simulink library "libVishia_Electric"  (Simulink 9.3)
settings: Solver=ode45  StartTime=0.0  StopTime=10.0  RelTol=1e-3  EnableMultiTasking=on
undefined symbols (not defined in the file or in its folder): C, Cp, Cs, ctRange, enable_Diode, fnom, gstart, Inom, Lline, n0, n2, nDamping, nHDamping, nIH, nIq, nLs, nPdamping, nRs, pWCstart, Rline, Rps, Rs, RsC, Tmech, Ts, TstepHw, Unom, xh
libraries: powerlib x111, libVishia_Conv x15, libVishia_Ctrl x6, $bdroot x2, lib_T1Blocks_FB x2, Lib_EnvA x1, lib_AngleBlocks x1
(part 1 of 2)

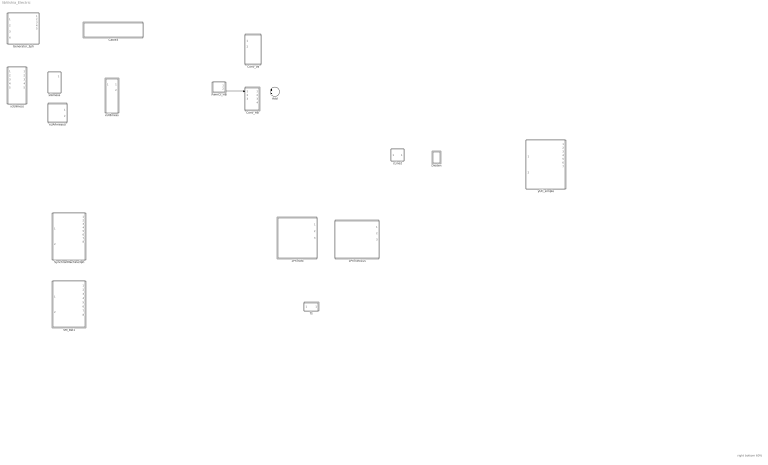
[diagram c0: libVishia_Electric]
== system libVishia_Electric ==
  note: right bottom 60%
  1PhTrafo : Subsystem
  1PhTrafo1us : Subsystem
  Add : Sum
  Cable3 : Subsystem
  Conv_HB : Subsystem
  Conv_Va : Subsystem
  Dioden : Subsystem
  Generator_3ph : Subsystem
  PwmCt_HB : Subsystem
  SM_Bel1 : Subsystem
  SynchronMachine3ph : Subsystem
  Ts : Subsystem
  cLine2 : Subsystem
  x3UImess : Subsystem
  xIAmess : Subsystem
  xUAFmeasU : Subsystem
  xUI3mess : Subsystem
  yUC_simple : Subsystem
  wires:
  PwmCt_HB/2(Out3) -> Conv_HB/1(In2)

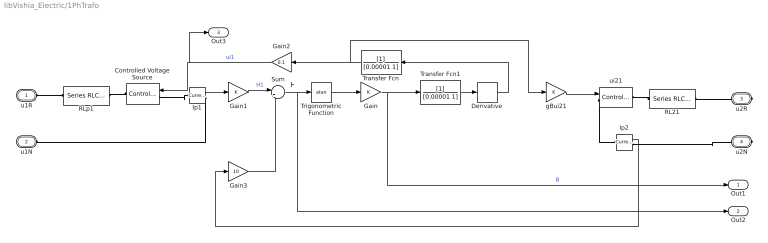
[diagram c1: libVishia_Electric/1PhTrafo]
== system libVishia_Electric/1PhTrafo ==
  note: H
  Controlled Voltage Source : powerlib/Electrical Sources/Controlled Voltage Source  Initialize=on  Source_Type=AC  Amplitude=0  Phase=0  Frequency=0  Measurements=None
  Derivative : Derivative
  Gain : Gain
  Gain1 : Gain
  Gain2 : Gain  Gain=0.1
  Gain3 : Gain  Gain=10
  Ip1 : powerlib/Measurements/Current Measurement  PhasorSimulation=off  OutputType=Complex  PSBequivalent=0
  Ip2 : powerlib/Measurements/Current Measurement  PhasorSimulation=off  OutputType=Complex  PSBequivalent=0
  RL21 : powerlib/Elements/Series RLC Branch  LConnTagsString=__new0  RConnTagsString=__new0  BranchType=RL  Resistance=1  Inductance=1e-3  SetiL0=off  InitialCurrent=0  Capacitance=1e-6  Setx0=off  InitialVoltage=0  Measurements=None
  RLp1 : powerlib/Elements/Series RLC Branch  LConnTagsString=__new0  RConnTagsString=__new0  BranchType=RL  Resistance=0.1  Inductance=0.0001  SetiL0=off  InitialCurrent=0  Capacitance=1e-6  Setx0=off  InitialVoltage=0  Measurements=None
  Sum : Sum  Inputs=|++
  Transfer Fcn : TransferFcn  Denominator=[0.00001 1]
  Transfer Fcn1 : TransferFcn  Denominator=[0.00001 1]
  Trigonometric Function : Trigonometry  Operator=atan
  gBui21 : Gain
  ui21 : powerlib/Electrical Sources/Controlled Voltage Source  Initialize=on  Source_Type=AC  Amplitude=0  Phase=0  Frequency=0  Measurements=None
  u1R : PMIOPort  Tag=PMCPort  Side=Left
  u1N : PMIOPort  Tag=PMCPort  Port=2  Side=Left
  u2R : PMIOPort  Tag=PMCPort  Port=3  Side=Right
  u2N : PMIOPort  Tag=PMCPort  Port=4  Side=Right
  Out1 : Outport
  Out2 : Outport  Port=2
  Out3 : Outport  Port=3
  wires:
  Trigonometric Function/1 -> Gain/1
  Gain/1 -> Transfer Fcn1/1, Out1/1  "B"
  gBui21/1 -> ui21/1
  Gain2/1 -> Out3/1, Controlled Voltage Source/1  "ui1"
  Derivative/1 -> Transfer Fcn/1
  Ip1/1 -> Gain1/1
  Transfer Fcn/1 -> gBui21/1, Gain2/1
  Gain1/1 -> Sum/1  "H1"
  Sum/1 -> Out2/1, Trigonometric Function/1
  Gain3/1 -> Sum/2
  Ip2/1 -> Gain3/1
  Transfer Fcn1/1 -> Derivative/1
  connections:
  u2R/RConn1 -- RL21/RConn1
  RLp1/RConn1 -- Controlled Voltage Source/RConn1
  Ip1/LConn1 -- Controlled Voltage Source/LConn1
  RLp1/LConn1 -- u1R/RConn1
  RL21/LConn1 -- ui21/RConn1
  Ip1/RConn1 -- u1N/RConn1
  ui21/LConn1 -- Ip2/LConn1
  u2N/RConn1 -- Ip2/RConn1

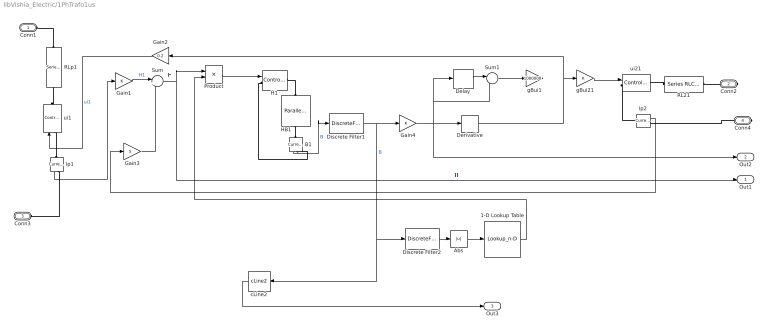
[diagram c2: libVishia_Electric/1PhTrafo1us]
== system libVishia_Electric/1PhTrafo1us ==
  note: H
  1-D Lookup Table : Lookup_n-D  NumberOfTableDimensions=1  BreakpointsForDimension1=[0 1 2 3 4 5]  Table="[1.0 0.9 0.7 0.3 0.15 0.05  ]"  InternalRulePriority=Speed  RndMeth=Simplest
  Abs : Abs
  B1 : powerlib/Measurements/Current Measurement  PhasorSimulation=off  OutputType=Complex  PSBequivalent=0
  Delay : Delay  DelayLength=1
  Derivative : Derivative
  Discrete Filter1 : DiscreteFilter  Denominator=[1 0.00001]
  Discrete Filter2 : DiscreteFilter  Denominator=[1 0.0001]
  Gain1 : Gain
  Gain2 : Gain  Gain=0.2
  Gain3 : Gain  Gain=5
  Gain4 : Gain
  H1 : powerlib/Electrical Sources/Controlled Voltage Source  Initialize=on  Source_Type=AC  Amplitude=0  Phase=0  Frequency=0  Measurements=None
  HB1 : powerlib/Elements/Parallel RLC Branch  LConnTagsString=a  RConnTagsString=__new0  BranchType=R  Resistance=1  Inductance=1e-3  SetiL0=off  InitialCurrent=0  Capacitance=1e-6  Setx0=off  InitialVoltage=0  Measurements=None
  Ip1 : powerlib/Measurements/Current Measurement  PhasorSimulation=off  OutputType=Complex  PSBequivalent=0
  Ip2 : powerlib/Measurements/Current Measurement  PhasorSimulation=off  OutputType=Complex  PSBequivalent=0
  Product : Product
  RL21 : powerlib/Elements/Series RLC Branch  LConnTagsString=__new0  RConnTagsString=__new0  BranchType=RL  Resistance=1  Inductance=1e-3  SetiL0=off  InitialCurrent=0  Capacitance=1e-6  Setx0=off  InitialVoltage=0  Measurements=None
  RLp1 : powerlib/Elements/Series RLC Branch  LConnTagsString=__new0  RConnTagsString=__new0  BranchType=RL  Resistance=0.1  Inductance=0.0001  SetiL0=off  InitialCurrent=0  Capacitance=1e-6  Setx0=off  InitialVoltage=0  Measurements=None
  Sum : Sum  Inputs=|++
  Sum1 : Sum  Inputs=|-+
  cLine2 : Lib_EnvA/cLine2  n0=1  xh=5  n2=0.05
  gBui1 : Gain  Gain=1000000
  gBui21 : Gain
  ui1 : powerlib/Electrical Sources/Controlled Voltage Source  Initialize=on  Source_Type=AC  Amplitude=0  Phase=0  Frequency=0  Measurements=None
  ui21 : powerlib/Electrical Sources/Controlled Voltage Source  Initialize=on  Source_Type=AC  Amplitude=0  Phase=0  Frequency=0  Measurements=None
  Conn1 : PMIOPort  Side=Left
  Conn2 : PMIOPort  Port=2  Side=Right
  Conn3 : PMIOPort  Port=3  Side=Left
  Conn4 : PMIOPort  Port=4  Side=Right
  Out1 : Outport
  Out2 : Outport  Port=2
  Out3 : Outport  Port=3
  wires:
  Abs/1 -> 1-D Lookup Table/1
  Discrete Filter2/1 -> Abs/1
  cLine2/1 -> Out3/1
  1-D Lookup Table/1 -> Product/2
  Gain4/1 -> Derivative/1, Out2/1, Sum1/2, Delay/1
  Gain2/1 -> ui1/1  "ui1"
  Ip2/1 -> Gain3/1
  Gain3/1 -> Sum/2
  Ip1/1 -> Gain1/1
  B1/1 -> Discrete Filter1/1  "B"
  gBui21/1 -> ui21/1
  Sum/1 -> Product/1, Out1/1  "H"
  Gain1/1 -> Sum/1  "H1"
  Sum1/1 -> gBui1/1
  Delay/1 -> Sum1/1
  Discrete Filter1/1 -> Gain4/1, cLine2/1, Discrete Filter2/1  "B"
  Derivative/1 -> Gain2/1, gBui21/1
  Product/1 -> H1/1
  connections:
  ui21/LConn1 -- Ip2/LConn1
  RLp1/RConn1 -- ui1/RConn1
  RLp1/LConn1 -- Conn1/RConn1
  Conn4/RConn1 -- Ip2/RConn1
  Ip1/RConn1 -- Conn3/RConn1
  RL21/RConn1 -- Conn2/RConn1
  RL21/LConn1 -- ui21/RConn1
  Ip1/LConn1 -- ui1/LConn1
  HB1/LConn1 -- H1/RConn1
  HB1/RConn1 -- B1/LConn1
  H1/LConn1 -- B1/RConn1

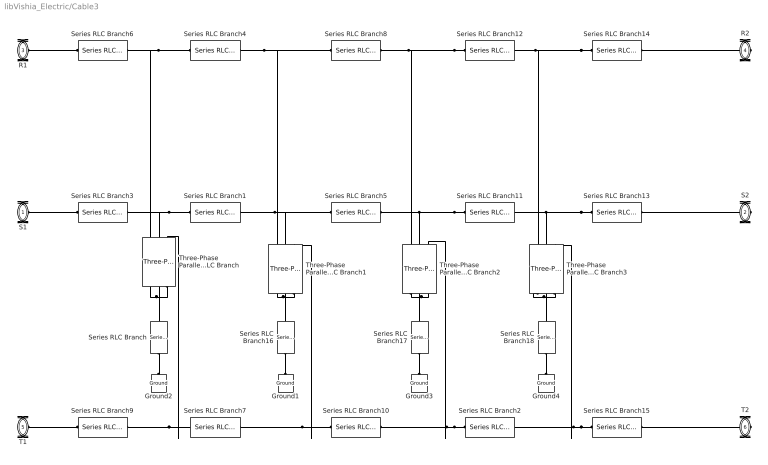
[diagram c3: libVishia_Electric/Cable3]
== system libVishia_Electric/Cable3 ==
  Ground{1..4} (4 alike) : powerlib/Elements/Ground  LConnTagsString=a
  Series RLC Branch{,16..18} (4 alike) : powerlib/Elements/Series RLC Branch  LConnTagsString=__new0  RConnTagsString=__new0  BranchType=R  Resistance=RsC  Inductance=1e-3  SetiL0=off  InitialCurrent=0  Capacitance=1e-6  Setx0=off  InitialVoltage=0  Measurements=None
  Series RLC Branch{1..2,4..5,7..8,10..12} (9 alike) : powerlib/Elements/Series RLC Branch  LConnTagsString=__new0  RConnTagsString=__new0  BranchType=RL  Resistance=Rline/4  Inductance=Lline/4  SetiL0=off  InitialCurrent=0  Capacitance=C  Setx0=off  InitialVoltage=0  Measurements=None
  Series RLC Branch{3,6,9,13..15} (6 alike) : powerlib/Elements/Series RLC Branch  LConnTagsString=__new0  RConnTagsString=__new0  BranchType=RL  Resistance=Rline/8  Inductance=Lline/8  SetiL0=off  InitialCurrent=0  Capacitance=C  Setx0=off  InitialVoltage=0  Measurements=None
  Three-Phase Parallel RLC Branch{,1..3} (4 alike) : powerlib/Elements/Three-Phase Parallel RLC Branch  LConnTagsString=A|B|C  RConnTagsString=A|B|C  BranchType=RC  Resistance=Rs/4  Inductance=1e-3  Capacitance=Cs/4  Measurements=None
  S1 : PMIOPort  Side=Left
  S2 : PMIOPort  Port=2  Side=Right
  R1 : PMIOPort  Port=3  Side=Left
  R2 : PMIOPort  Port=4  Side=Right
  T1 : PMIOPort  Port=5  Side=Left
  T2 : PMIOPort  Port=6  Side=Right
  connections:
  Three-Phase Parallel RLC Branch2/RConn1 -- Three-Phase Parallel RLC Branch2/RConn2 -- Series RLC Branch17/LConn1 -- Three-Phase Parallel RLC Branch2/RConn3
  S1/RConn1 -- Series RLC Branch3/RConn1
  Series RLC Branch1/RConn1 -- Three-Phase Parallel RLC Branch/LConn2 -- Series RLC Branch3/LConn1
  Series RLC Branch4/RConn1 -- Three-Phase Parallel RLC Branch/LConn1 -- Series RLC Branch6/LConn1
  R1/RConn1 -- Series RLC Branch6/RConn1
  Series RLC Branch9/LConn1 -- Three-Phase Parallel RLC Branch/LConn3 -- Series RLC Branch7/RConn1
  T1/RConn1 -- Series RLC Branch9/RConn1
  Series RLC Branch4/LConn1 -- Three-Phase Parallel RLC Branch1/LConn1 -- Series RLC Branch8/RConn1
  Series RLC Branch1/LConn1 -- Three-Phase Parallel RLC Branch1/LConn2 -- Series RLC Branch5/RConn1
  Series RLC Branch7/LConn1 -- Three-Phase Parallel RLC Branch1/LConn3 -- Series RLC Branch10/RConn1
  Series RLC Branch12/RConn1 -- Series RLC Branch8/LConn1 -- Three-Phase Parallel RLC Branch2/LConn1
  Series RLC Branch11/RConn1 -- Series RLC Branch5/LConn1 -- Three-Phase Parallel RLC Branch2/LConn2
  Series RLC Branch2/RConn1 -- Series RLC Branch10/LConn1 -- Three-Phase Parallel RLC Branch2/LConn3
  Series RLC Branch14/RConn1 -- Series RLC Branch12/LConn1 -- Three-Phase Parallel RLC Branch3/LConn1
  Series RLC Branch13/RConn1 -- Series RLC Branch11/LConn1 -- Three-Phase Parallel RLC Branch3/LConn2
  Series RLC Branch15/RConn1 -- Series RLC Branch2/LConn1 -- Three-Phase Parallel RLC Branch3/LConn3
  R2/RConn1 -- Series RLC Branch14/LConn1
  S2/RConn1 -- Series RLC Branch13/LConn1
  T2/RConn1 -- Series RLC Branch15/LConn1
  Three-Phase Parallel RLC Branch/RConn3 -- Series RLC Branch/LConn1 -- Three-Phase Parallel RLC Branch/RConn1 -- Three-Phase Parallel RLC Branch/RConn2
  Three-Phase Parallel RLC Branch1/RConn3 -- Series RLC Branch16/LConn1 -- Three-Phase Parallel RLC Branch1/RConn1 -- Three-Phase Parallel RLC Branch1/RConn2
  Three-Phase Parallel RLC Branch3/RConn3 -- Three-Phase Parallel RLC Branch3/RConn2 -- Series RLC Branch18/LConn1 -- Three-Phase Parallel RLC Branch3/RConn1
  Series RLC Branch/RConn1 -- Ground2/LConn1
  Series RLC Branch16/RConn1 -- Ground1/LConn1
  Series RLC Branch17/RConn1 -- Ground3/LConn1
  Series RLC Branch18/RConn1 -- Ground4/LConn1

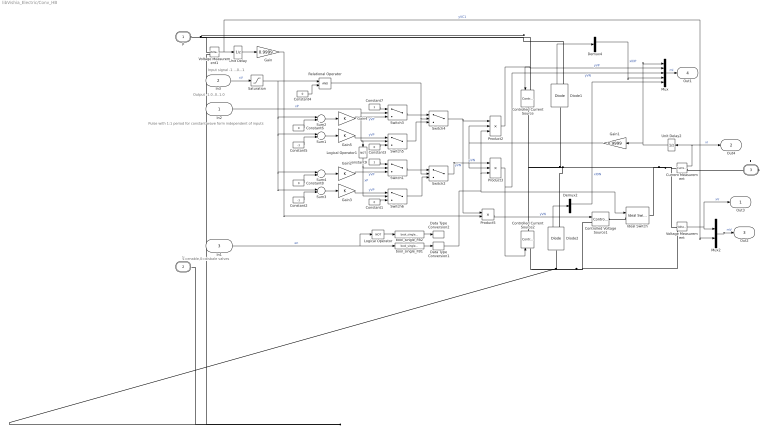
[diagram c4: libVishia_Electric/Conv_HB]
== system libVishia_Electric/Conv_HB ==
  note: Pulse with 1:1 period for constant wave form independent of inputs
  note: Input signal -1 ...0...1
  note: 1=enable,0=disbale valves
  note: Output -1.0..0..1.0
  In2 : Inport
  In3 : Inport  Port=2  OutDataTypeStr=single
  In1 : Inport  Port=3
  Constant{1,3..4,6,8} (5 alike) : Constant  Value=0
  Constant2 : Constant  Value=-1
  Constant5 : Constant  Value=-1
  Constant7 : Constant
  Constant9 : Constant
  Controlled Current Source : powerlib/Electrical Sources/Controlled Current Source  Initialize=on  Source_Type=AC  Amplitude=0  Phase=0  Frequency=0  Measurements=None
  Controlled Current Source2 : powerlib/Electrical Sources/Controlled Current Source  Initialize=on  Source_Type=AC  Amplitude=0  Phase=0  Frequency=0  Measurements=None
  Controlled Voltage Source1 : powerlib/Electrical Sources/Controlled Voltage Source  Initialize=on  Source_Type=AC  Amplitude=0  Phase=0  Frequency=0  Measurements=None
  Current Measurement : powerlib/Measurements/Current Measurement  PhasorSimulation=off  OutputType=Complex  PSBequivalent=0
  Data Type Conversion1 : DataTypeConversion  OutDataTypeStr=double
  Data Type Conversion2 : DataTypeConversion  OutDataTypeStr=double
  Demux2 : Demux  Outputs=2
  Demux4 : Demux  Outputs=2
  Diode1 : powerlib/Power Electronics/Diode  Ron=0.001  Lon=0  Vf=0.8  IC=0  UseSnubber=0  Rs=500  Cs=250e-9  Measurements=on
  Diode2 : powerlib/Power Electronics/Diode  Ron=0.001  Lon=0  Vf=0.8  IC=0  UseSnubber=0  Rs=500  Cs=250e-9  Measurements=on
  Gain : Gain  Gain=0.9999
  Gain1 : Gain  Gain=0.9999
  Gain{2..5} (4 alike) : Gain
  Ideal Switch : powerlib/Power Electronics/Ideal Switch  Ron=0.001  Lon=0  IC=0  Rs=1e5  Cs=inf  Measurements=off
  Logical Operator : Logic  Operator=NOT  IconShape=distinctive  AllPortsSameDT=off  OutDataTypeStr=boolean
  Logical Operator1 : Logic  Operator=NOT  IconShape=distinctive  AllPortsSameDT=off  OutDataTypeStr=boolean
  Mux : Mux  Inputs=5
  Mux2 : Mux  Inputs=2
  Product2 : Product  Inputs=3
  Product3 : Product  Inputs=3
  Product5 : Product
  Relational Operator : RelationalOperator  OutDataTypeStr=boolean  RndMeth=Simplest
  Saturation : Saturate  UpperLimit=1.0  LowerLimit=-1.0
  Sum{1..4} (4 alike) : Sum  Inputs=|+-
  Switch{1..6} (6 alike) : Switch  Criteria=u2 ~= 0
  Unit Delay : UnitDelay  SampleTime=-1  HasFrameUpgradeWarning=on
  Unit Delay2 : UnitDelay  SampleTime=-1  HasFrameUpgradeWarning=on
  Voltage Measurement : powerlib/Measurements/Voltage Measurement  PhasorSimulation=off  OutputType=Complex  PSBequivalent=0
  Voltage Measurement1 : powerlib/Measurements/Voltage Measurement  PhasorSimulation=off  OutputType=Complex  PSBequivalent=0
  bool_single_FB1 : libVishia_Conv/bool_single_FB  hi=1  lo=0
  bool_single_FB2 : libVishia_Conv/bool_single_FB  hi=1  lo=0
  P : PMIOPort  Tag=PMCPort  Side=Left
  N : PMIOPort  Tag=PMCPort  Port=2  Side=Left
  L : PMIOPort  Tag=PMCPort  Port=3  Side=Right
  Out3 : Outport  OutDataTypeStr=double
  Out4 : Outport  Port=2  OutDataTypeStr=double
  Out2 : Outport  Port=3  OutDataTypeStr=double
  Out1 : Outport  Port=4  OutDataTypeStr=double
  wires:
  Diode2/1 -> Demux2/1
  Diode1/1 -> Demux4/1
  Data Type Conversion1/1 -> Product2/3, Product3/3, Ideal Switch/1
  bool_single_FB1/1 -> Data Type Conversion1/1
  In1/1 -> Logical Operator/1, bool_single_FB1/1  "en"
  Switch3/1 -> Switch4/1
  Constant7/1 -> Switch3/1
  Switch4/1 -> Product5/1, Product2/1  "yVN"
  Sum2/1 -> Gain4/1
  Constant6/1 -> Sum2/2
  Constant5/1 -> Sum1/2
  Sum1/1 -> Gain5/1
  Constant4/1 -> Relational Operator/2
  Relational Operator/1 -> Switch2/2, Switch4/2
  Switch5/1 -> Switch4/3
  Constant3/1 -> Switch5/3
  Gain5/1 -> Switch5/1  "yVP"
  Gain4/1 -> Switch3/3  "yVP"
  Product3/1 -> Controlled Current Source2/1, Mux/3  "yVN"
  Product2/1 -> Controlled Current Source/1, Mux/2  "yVP"
  Product5/1 -> Controlled Voltage Source1/1  "yVN"
  Voltage Measurement1/1 -> Unit Delay/1, Mux2/2  "yVC1"
  In2/1 -> Logical Operator1/1, Switch5/2, Switch3/2  "xP"
  Gain/1 -> Product5/2
  Demux4/1 -> Mux/4  "xIDP"
  Demux2/1 -> Mux/5  "xIDN"
  Mux/1 -> Out1/1  "mI"
  Mux2/1 -> Out2/1  "mV"
  Current Measurement/1 -> Out4/1, Unit Delay2/1  "xI"
  Voltage Measurement/1 -> Out3/1, Mux2/1  "xV"
  Gain1/1 -> Product2/2, Product3/2
  Unit Delay2/1 -> Mux/1, Gain1/1
  Unit Delay/1 -> Gain/1
  bool_single_FB2/1 -> Data Type Conversion2/1
  Logical Operator/1 -> bool_single_FB2/1
  In3/1 -> Saturation/1  "xV"
  Constant2/1 -> Sum3/2
  Constant1/1 -> Switch6/3
  Logical Operator1/1 -> Switch1/2, Switch6/2  "xP"
  Gain2/1 -> Switch1/3  "yVP"
  Sum3/1 -> Gain3/1
  Constant8/1 -> Sum4/2
  Switch1/1 -> Switch2/1
  Sum4/1 -> Gain2/1
  Constant9/1 -> Switch1/1
  Switch6/1 -> Switch2/3
  Gain3/1 -> Switch6/1  "yVP"
  Switch2/1 -> Product3/1  "yVN"
  Saturation/1 -> Sum3/1, Sum4/1, Sum1/1, Sum2/1, Relational Operator/1
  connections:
  Ideal Switch/LConn1 -- Controlled Voltage Source1/RConn1
  Controlled Current Source/LConn1 -- Diode1/RConn1 -- P/RConn1 -- Voltage Measurement1/LConn1
  Controlled Current Source2/LConn1 -- N/RConn1 -- Voltage Measurement1/LConn2 -- Diode2/LConn1 -- Controlled Voltage Source1/LConn1 -- Voltage Measurement/LConn2
  Voltage Measurement/LConn1 -- Current Measurement/LConn1 -- Ideal Switch/RConn1 -- Diode1/LConn1 -- Controlled Current Source/RConn1 -- Controlled Current Source2/RConn1 -- Diode2/RConn1
  Current Measurement/RConn1 -- L/RConn1

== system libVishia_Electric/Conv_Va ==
  In1 : Inport
  In2 : Inport  Port=2
  Diode2 : powerlib/Power Electronics/Diode  Ron=0.001  Lon=0  Vf=0.8  IC=0  UseSnubber=0  Rs=500  Cs=250e-9  Measurements=on
  Diode3 : powerlib/Power Electronics/Diode  Ron=0.001  Lon=0  Vf=0.8  IC=0  UseSnubber=0  Rs=500  Cs=250e-9  Measurements=on
  Ideal Switch : powerlib/Power Electronics/Ideal Switch  Ron=0.001  Lon=0  IC=0  Rs=1e5  Cs=inf  Measurements=on
  Ideal Switch1 : powerlib/Power Electronics/Ideal Switch  Ron=0.001  Lon=0  IC=0  Rs=1e5  Cs=inf  Measurements=on
  Series RLC Branch : powerlib/Elements/Series RLC Branch  LConnTagsString=__new0  RConnTagsString=__new0  BranchType=RC  Resistance=Rps  Inductance=1e-3  SetiL0=off  InitialCurrent=0  Capacitance=Cp  Setx0=off  InitialVoltage=0  Measurements=None
  Series RLC Branch1 : powerlib/Elements/Series RLC Branch  LConnTagsString=__new0  RConnTagsString=__new0  BranchType=RC  Resistance=Rps  Inductance=1e-3  SetiL0=off  InitialCurrent=0  Capacitance=Cp  Setx0=off  InitialVoltage=0  Measurements=None
  bool2single1 : libVishia_Conv/bool_single_FB  hi=1.0  lo=0
  bool2single3 : libVishia_Conv/bool_single_FB  hi=1.0  lo=0
  P : PMIOPort  Tag=PMCPort  Side=Left
  N : PMIOPort  Tag=PMCPort  Port=2  Side=Left
  L : PMIOPort  Tag=PMCPort  Port=3  Side=Right
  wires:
  In1/1 -> bool2single3/1  "H"
  In2/1 -> bool2single1/1  "L"
  bool2single3/1 -> Ideal Switch/1
  bool2single1/1 -> Ideal Switch1/1
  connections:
  Ideal Switch/RConn1 -- Series RLC Branch1/LConn1 -- L/RConn1 -- Series RLC Branch/RConn1 -- Diode3/RConn1 -- Diode2/LConn1 -- Ideal Switch1/LConn1
  N/RConn1 -- Series RLC Branch1/RConn1 -- Diode3/LConn1 -- Ideal Switch1/RConn1
  P/RConn1 -- Series RLC Branch/LConn1 -- Diode2/RConn1 -- Ideal Switch/LConn1

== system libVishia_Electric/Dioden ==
  Breaker : powerlib/Elements/Breaker  InitialState=0  SwitchingTimes="[ 1/60  5/60 ]"  External=on  BreakerResistance=0.0000001  SnubberResistance=inf  SnubberCapacitance=1e-6  Measurements=None  MoreParameters=off  NoBreakLoop=off
  Constant : Constant  Value=enable_Diode  OutDataTypeStr=int32
  Diode : powerlib/Power Electronics/Diode  Ron=0.0001  Lon=0  Vf=Vf_Diode  IC=0  UseSnubber=off  Rs=inf  Cs=0  Measurements=off
  Diode3 : powerlib/Power Electronics/Diode  Ron=0.0001  Lon=0  Vf=Vf_Diode  IC=0  UseSnubber=off  Rs=inf  Cs=0  Measurements=off
  Logical Operator : Logic  Operator=NOT  AllPortsSameDT=off  OutDataTypeStr=boolean
  Series RLC Branch : powerlib/Elements/Series RLC Branch  LConnTagsString=__new0  RConnTagsString=__new0  BranchType=R  Resistance=10000  Inductance=1e-3  SetiL0=off  InitialCurrent=0  Capacitance=1e-6  Setx0=off  InitialVoltage=0  Measurements=None
  in : PMIOPort  Tag=PMCPort  Side=Left
  out : PMIOPort  Tag=PMCPort  Port=2  Side=Right
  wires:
  Logical Operator/1 -> Breaker/1
  Constant/1 -> Logical Operator/1
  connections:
  Series RLC Branch/LConn1 -- Diode3/RConn1 -- in/RConn1 -- Breaker/LConn1 -- Diode/LConn1
  Series RLC Branch/RConn1 -- Diode/RConn1 -- out/RConn1 -- Breaker/RConn1 -- Diode3/LConn1

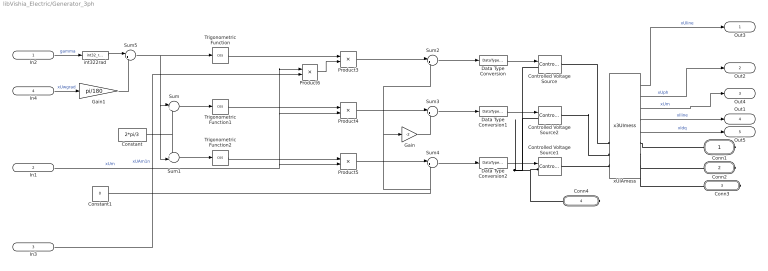
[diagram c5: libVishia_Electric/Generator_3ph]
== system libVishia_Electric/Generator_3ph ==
  In2 : Inport  OutDataTypeStr=int32
  In1 : Inport  Port=2  OutDataTypeStr=single  PortDimensions=1
  In3 : Inport  Port=3  OutDataTypeStr=single  PortDimensions=1
  In4 : Inport  Port=4  OutDataTypeStr=single  PortDimensions=1
  Constant : Constant  Value=2*pi/3  OutDataTypeStr=single
  Constant1 : Constant  Value=0
  Controlled Voltage Source : powerlib/Electrical Sources/Controlled Voltage Source  Initialize=on  Source_Type=AC  Amplitude=0  Phase=0  Frequency=0  Measurements=None
  Controlled Voltage Source1 : powerlib/Electrical Sources/Controlled Voltage Source  Initialize=on  Source_Type=AC  Amplitude=0  Phase=0  Frequency=0  Measurements=None
  Controlled Voltage Source2 : powerlib/Electrical Sources/Controlled Voltage Source  Initialize=on  Source_Type=AC  Amplitude=0  Phase=0  Frequency=0  Measurements=None
  Data Type Conversion : DataTypeConversion
  Data Type Conversion1 : DataTypeConversion
  Data Type Conversion2 : DataTypeConversion
  Gain : Gain  Gain=-2
  Gain1 : Gain  Gain=pi/180
  Product{3..6} (4 alike) : Product
  Sum : Sum  Inputs=|+-
  Sum1 : Sum  Inputs=++|
  Sum{2..5} (4 alike) : Sum  Inputs=|++
  Trigonometric Function : Trigonometry  Operator=cos
  Trigonometric Function1 : Trigonometry  Operator=cos
  Trigonometric Function2 : Trigonometry  Operator=cos
  int322rad : libVishia_Conv/int32_rad_FB  SystemSampleTime=-1
  xUIAmess : $bdroot/x3UImess  SystemSampleTime=-1
  Conn1 : PMIOPort  Side=Right
  Conn2 : PMIOPort  Port=2  Side=Right
  Conn3 : PMIOPort  Port=3  Side=Right
  Conn4 : PMIOPort  Port=4  Side=Right
  Out3 : Outport  OutDataTypeStr=single  PortDimensions=3
  Out2 : Outport  Port=2  OutDataTypeStr=single  PortDimensions=3
  Out4 : Outport  Port=3  OutDataTypeStr=single  PortDimensions=1
  Out1 : Outport  Port=4  OutDataTypeStr=single  PortDimensions=3
  Out5 : Outport  Port=5  OutDataTypeStr=single  PortDimensions=1
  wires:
  Constant/1 -> Sum1/1, Sum/2
  Sum1/1 -> Trigonometric Function2/1
  Sum/1 -> Trigonometric Function1/1
  Sum5/1 -> Sum1/2, Sum/1, Trigonometric Function/1
  In2/1 -> int322rad/1  "gamma"
  Data Type Conversion/1 -> Controlled Voltage Source/1
  Data Type Conversion1/1 -> Controlled Voltage Source2/1
  Data Type Conversion2/1 -> Controlled Voltage Source1/1
  Product4/1 -> Sum3/1
  Product3/1 -> Sum2/1
  In1/1 -> Product6/1, Product4/2, Product5/2  "xUm"
  Product5/1 -> Sum4/1
  Trigonometric Function/1 -> Product3/1
  Trigonometric Function1/1 -> Product4/1
  Trigonometric Function2/1 -> Product5/1
  Sum2/1 -> Data Type Conversion/1
  Sum3/1 -> Data Type Conversion1/1
  Sum4/1 -> Data Type Conversion2/1
  Constant1/1 -> Gain/1, Sum2/2, Sum4/2
  Gain/1 -> Sum3/2
  Product6/1 -> Product3/2
  In3/1 -> Product6/2  "xUAm1n"
  int322rad/1 -> Sum5/1
  In4/1 -> Gain1/1  "xUwgrad"
  Gain1/1 -> Sum5/2
  xUIAmess/2 -> Out2/1  "xUph"
  xUIAmess/1 -> Out3/1  "xUline"
  xUIAmess/4 -> Out1/1  "xIline"
  xUIAmess/3 -> Out4/1  "xUm"
  xUIAmess/5 -> Out5/1  "xIdq"
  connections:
  Controlled Voltage Source1/LConn1 -- Conn4/RConn1 -- Controlled Voltage Source/LConn1 -- Controlled Voltage Source2/LConn1
  xUIAmess/LConn1 -- Controlled Voltage Source/RConn1
  xUIAmess/LConn2 -- Controlled Voltage Source2/RConn1
  xUIAmess/LConn3 -- Controlled Voltage Source1/RConn1
  xUIAmess/RConn3 -- Conn3/RConn1
  xUIAmess/RConn2 -- Conn2/RConn1
  xUIAmess/RConn1 -- Conn1/RConn1

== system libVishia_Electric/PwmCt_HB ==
  note: counts from 0 t0 ctRange-1 ctRange should be even (able to divide by 2)
  Constant3 : Constant  Value=0  OutDataTypeStr=int16
  Constant4 : Constant  Value=ctRange-1  OutDataTypeStr=int16
  Constant5 : Constant  OutDataTypeStr=int16
  Constant6 : Constant  Value=ctRange/2  OutDataTypeStr=int16
  Relational Operator2 : RelationalOperator  OutDataTypeStr=boolean  RndMeth=Simplest
  Relational Operator7 : RelationalOperator  OutDataTypeStr=boolean  RndMeth=Simplest
  addS_OpC : libVishia_Ctrl/addS_OpC  init=0  Tstep=-1
  Out2 : Outport  OutDataTypeStr=int16
  Out3 : Outport  Port=2  OutDataTypeStr=boolean
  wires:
  Relational Operator7/1 -> addS_OpC/3
  addS_OpC/2 -> Relational Operator2/1, Relational Operator7/1, Out2/1  "yCt"
  Constant6/1 -> Relational Operator2/2
  Constant4/1 -> Relational Operator7/2
  Constant3/1 -> addS_OpC/2
  Constant5/1 -> addS_OpC/1
  Relational Operator2/1 -> Out3/1  "yP"

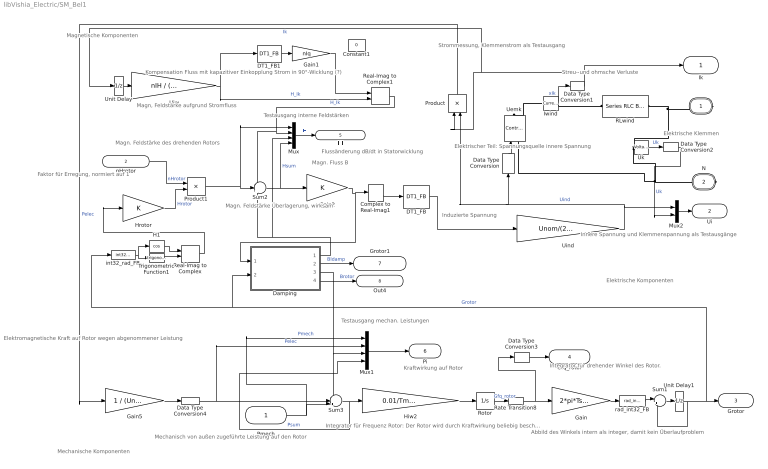
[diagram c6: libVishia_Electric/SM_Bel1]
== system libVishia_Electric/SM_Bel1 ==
  note: Abbild des Winkels intern als integer, damit kein Überlaufproblem
  note: Kompensation Fluss mit kapazitiver Einkopplung Strom in 90°-Wicklung (?)
  note: Testausgang mechan. Leistungen
  note: Mechanische Komponenten
  note: Mechanisch von außen zugeführte Leistung auf den Rotor
  note: Elektromagnetische Kraft auf Rotor wegen abgenommener Leistung
  note: Strommessung, Klemmenstrom als Testausgang
  note: Innere Spannung und Klemmenspannung als Testausgänge
  note: Elektrische Klemmen
  note: Streu- und ohmsche Verluste
  note: Elektrischer Teil: Spannungsquelle innere Spannung
  note: Faktor für Erregung, normiert auf 1
  note: Testausgang interne Feldstärken
  note: Flussänderung dB/dt in Statorwicklung
  note: Magn. Fluss B
  note: Induzierte Spannung
  note: Magn, Feldstärke aufgrund Stromfluss
  note: Magn. Feldstärke Überlagerung, wirksam
  note: Integrator für Frequenz Rotor: Der Rotor wird durch Kraftwirkung beliebig beschleunigt. Reibungsverluste hier unberücksichtigt.
  note: Kraftwirkung auf Rotor
  note: Integrator für drehender Winkel des Rotor.
  note: Magn. Feldstärke des drehenden Rotors
  note: Magnetische Komponenten
  note: Elektrische Komponenten
  Pmech : Inport  OutDataTypeStr=double  PortDimensions=1
  nHrotor : Inport  Port=2  OutDataTypeStr=single  PortDimensions=1
  Complex to Real-Imag1 : ComplexToRealImag
  Constant1 : Constant  Value=0  OutDataTypeStr=single
  DT1_FB : libVishia_Ctrl/DT1_FB  T1=0.0004  Td=1  Tstep=TstepHw
  DT1_FB1 : libVishia_Ctrl/DT1_FB  T1=0.001  Td=0.060/2/pi  Tstep=TstepHw
  Damping : Subsystem
  Data Type Conversion : DataTypeConversion  OutDataTypeStr=double
  Data Type Conversion1 : DataTypeConversion  OutDataTypeStr=single
  Data Type Conversion2 : DataTypeConversion  OutDataTypeStr=single
  Data Type Conversion3 : DataTypeConversion  OutDataTypeStr=single
  Data Type Conversion4 : DataTypeConversion  OutDataTypeStr=double
  Gain : Gain  Gain=2*pi*TstepHw
  Gain1 : Gain  Gain=nIq
  Gain2 : Gain
  Gain5 : Gain  Gain=1 / (Unom*Inom)
  H1 : Trigonometry  Operator=cos
  Hiw : Gain  Gain=nIH / (Inom*sqrt(2))
  Hiw2 : Gain  Gain=0.01/Tmech
  Hrotor : Gain
  Iwind : powerlib/Measurements/Current Measurement  PhasorSimulation=off  OutputType=Complex  PSBequivalent=0
  Mux : Mux
  Mux1 : Mux
  Mux2 : Mux  Inputs=2
  Product : Product
  Product1 : Product
  RLwind : powerlib/Elements/Series RLC Branch  LConnTagsString=__new0  RConnTagsString=__new0  BranchType=RL  Resistance=nRs*Unom/Inom  Inductance=nLs * Unom/Inom / (2*pi*fnom)  SetiL0=off  InitialCurrent=0  Capacitance=1e-6  Setx0=off  InitialVoltage=0  Measurements=None
  Rate Transition8 : RateTransition  Integrity=off  Deterministic=off  OutPortSampleTimeMultiple=16  OutPortSampleTime=TstepHw
  Real-Imag to Complex : RealImagToComplex
  Real-Imag to Complex1 : RealImagToComplex
  Rotor : Integrator  InitialCondition=fnom
  Sum1 : Sum  Inputs=|++
  Sum2 : Sum  Inputs=-++
  Sum3 : Sum  Inputs=--+
  Trigonometric Function1 : Trigonometry
  Uemk : powerlib/Electrical Sources/Controlled Voltage Source  Initialize=on  Source_Type=AC  Amplitude=0  Phase=0  Frequency=0  Measurements=None
  Uind : Gain  Gain=Unom/(2*pi*fnom)*sqrt(2)
  Uk : powerlib/Measurements/Voltage Measurement  PhasorSimulation=off  OutputType=Complex  PSBequivalent=0
  Unit Delay : UnitDelay  SampleTime=-1  HasFrameUpgradeWarning=on
  Unit Delay1 : UnitDelay  InitialCondition=gstart*65536*32768/180  SampleTime=TstepHw  HasFrameUpgradeWarning=on
  int32_rad_FB : libVishia_Conv/int32_rad_FB  SystemSampleTime=-1
  rad_int32_FB : libVishia_Conv/rad_int32_FB  SystemSampleTime=-1
  L : PMIOPort  Tag=PMCPort  Side=Right
  N : PMIOPort  Tag=PMCPort  Port=2  Side=Right
  Ik : Outport  OutDataTypeStr=single  PortDimensions=1
  Ui : Outport  Port=2  PortDimensions=2
  Grotor : Outport  Port=3  OutDataTypeStr=int32  PortDimensions=1
  Gfq_rotor : Outport  Port=4  PortDimensions=1
  Hi : Outport  Port=5  PortDimensions=4
  Pi : Outport  Port=6  OutDataTypeStr=double  PortDimensions=4
  Grotor1 : Outport  Port=7  OutDataTypeStr=single  PortDimensions=3
  Out4 : Outport  Port=8  OutDataTypeStr=single  PortDimensions=1
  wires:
  Damping/2(Out2) -> Grotor1/1  "BIdamp"
  Damping/1(Out1) -> Sum2/3, Mux/3
  Hrotor/1 -> Product1/2  "Hrotor"
  nHrotor/1 -> Product1/1  "nHrotor"
  DT1_FB/2 -> Uind/1
  Hiw2/1 -> Rotor/1
  Data Type Conversion3/1 -> Gfq_rotor/1
  Rate Transition8/1 -> Gain/1, Data Type Conversion3/1
  Mux1/1 -> Pi/1
  Real-Imag to Complex/1 -> Hrotor/1
  Mux2/1 -> Ui/1
  Product/1 -> Gain5/1  "Pelec"
  Data Type Conversion4/1 -> Mux1/2, Sum3/2  "Pelec"
  Sum3/1 -> Mux1/4, Hiw2/1  "Psum"
  Unit Delay/1 -> Hiw/1
  Uk/1 -> Data Type Conversion2/1  "Uk"
  Data Type Conversion2/1 -> Mux2/2  "Uk"
  Data Type Conversion1/1 -> Ik/1, Product/1, Unit Delay/1  "Ik"
  Mux/1 -> Hi/1  "Hi"
  Real-Imag to Complex1/1 -> Sum2/1, Mux/2  "H_Ik"
  Uind/1 -> Data Type Conversion/1, Product/2, Mux2/1  "Uind"
  Sum2/1 -> Mux/4, Gain2/1  "Hsum"
  Iwind/1 -> Data Type Conversion1/1  "xIk"
  Data Type Conversion/1 -> Uemk/1
  Rotor/1 -> Rate Transition8/1  "Gfq_rotor"
  rad_int32_FB/1 -> Sum1/1
  Gain/1 -> rad_int32_FB/1
  Unit Delay1/1 -> Sum1/2, Grotor/1, Damping/2(In3), int32_rad_FB/1  "Grotor"
  Sum1/1 -> Unit Delay1/1
  Pmech/1 -> Sum3/3, Mux1/1  "Pmech"
  Gain5/1 -> Data Type Conversion4/1
  Product1/1 -> Sum2/2, Mux/1
  Gain2/1 -> Complex to Real-Imag1/1, Damping/1(In1)
  Trigonometric Function1/1 -> Real-Imag to Complex/2
  H1/1 -> Real-Imag to Complex/1
  int32_rad_FB/1 -> Trigonometric Function1/1, H1/1
  Gain1/1 -> Real-Imag to Complex1/1
  Hiw/1 -> Real-Imag to Complex1/2, DT1_FB1/1  "H_Ik"
  Complex to Real-Imag1/2 -> DT1_FB/1
  Damping/3(Out3) -> Sum3/1, Mux1/3
  Damping/4(Out4) -> Out4/1  "Brotor"
  DT1_FB1/2 -> Gain1/1
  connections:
  Iwind/LConn1 -- Uemk/RConn1
  Uk/LConn1 -- RLwind/RConn1 -- L/RConn1
  Iwind/RConn1 -- RLwind/LConn1
  Uk/LConn2 -- Uemk/LConn1 -- N/RConn1

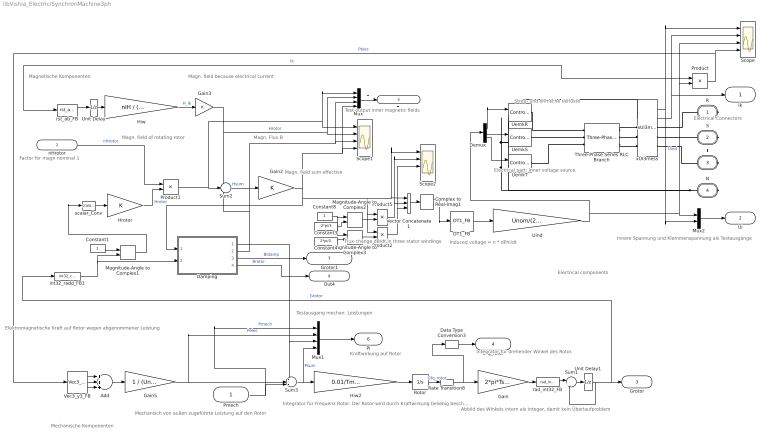
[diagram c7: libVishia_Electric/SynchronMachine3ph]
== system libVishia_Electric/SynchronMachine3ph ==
  note: Electrical components
  note: Magnetische Komponenten
  note: Magn. field of rotating rotor
  note: Integrator für drehender Winkel des Rotor.
  note: Kraftwirkung auf Rotor
  note: Integrator für Frequenz Rotor: Der Rotor wird durch Kraftwirkung beliebig beschleunigt. Reibungsverluste hier unberücksichtigt.
  note: Magn. field sum effective
  note: Magn. field because electrical current
  note: Induced voltage = n * dPhi/dt
  note: Magn. Flux B
  note: Flux-change dB/dt in three stator windings
  note: Test output inner magnetic fields
  note: Factor for magn nominal 1
  note: Electrical part: inner voltage source
  note: Streu- und ohmsche Verluste
  note: Electrical Connectors
  note: Innere Spannung und Klemmenspannung als Testausgänge
  note: Elektromagnetische Kraft auf Rotor wegen abgenommener Leistung
  note: Mechanisch von außen zugeführte Leistung auf den Rotor
  note: Mechanische Komponenten
  note: Testausgang mechan. Leistungen
  note: Abbild des Winkels intern als integer, damit kein Überlaufproblem
  Pmech : Inport  OutDataTypeStr=double  PortDimensions=1
  nHrotor : Inport  Port=2  OutDataTypeStr=double  PortDimensions=1
  Add : Sum  Inputs=+++
  Complex to Real-Imag1 : ComplexToRealImag
  Constant1 : Constant  OutDataTypeStr=double
  Constant3 : Constant  Value=-2*pi/3  OutDataTypeStr=double
  Constant4 : Constant  Value=2*pi/3  OutDataTypeStr=double
  Constant8 : Constant  OutDataTypeStr=double
  DT1_FB : libVishia_Ctrl/DT1_FB  T1=0.0004  Td=1  Tstep=TstepHw
  Damping : Subsystem
  Data Type Conversion3 : DataTypeConversion  OutDataTypeStr=single
  Demux : Demux  Outputs=3
  Gain : Gain  Gain=2*pi*TstepHw
  Gain2 : Gain
  Gain3 : Gain
  Gain5 : Gain  Gain=1 / (Unom*Inom)
  Hiw : Gain  Gain=nIH / (Inom*sqrt(2))
  Hiw2 : Gain  Gain=0.01/Tmech
  Hrotor : Gain
  Magnitude-Angle to Complex1 : MagnitudeAngleToComplex
  Magnitude-Angle to Complex2 : MagnitudeAngleToComplex
  Magnitude-Angle to Complex3 : MagnitudeAngleToComplex
  Mux : Mux
  Mux1 : Mux
  Mux2 : Mux  Inputs=2
  Product{,1..2,5} (4 alike) : Product
  Rate Transition8 : RateTransition  Integrity=off  Deterministic=off  OutPortSampleTimeMultiple=16  OutPortSampleTime=TstepHw
  Rotor : Integrator  InitialCondition=fnom
  Scope : Scope  NumInputPorts=4
  Scope1 : Scope  NumInputPorts=4
  Scope2 : Scope  NumInputPorts=4
  Sum1 : Sum  Inputs=|++
  Sum2 : Sum  Inputs=-+-
  Sum3 : Sum  Inputs=+-+
  Three-Phase Series RLC Branch : powerlib/Elements/Three-Phase Series RLC Branch  LConnTagsString=A|B|C  RConnTagsString=A|B|C  BranchType=RL  Resistance=nRs*Unom/Inom  Inductance=nLs * Unom/Inom / (2*pi*fnom)  Capacitance=1e-6  Measurements=None
  UemkR : powerlib/Electrical Sources/Controlled Voltage Source  Initialize=on  Source_Type=AC  Amplitude=0  Phase=0  Frequency=0  Measurements=None
  UemkS : powerlib/Electrical Sources/Controlled Voltage Source  Initialize=on  Source_Type=AC  Amplitude=0  Phase=0  Frequency=0  Measurements=None
  UemkT : powerlib/Electrical Sources/Controlled Voltage Source  Initialize=on  Source_Type=AC  Amplitude=0  Phase=0  Frequency=0  Measurements=None
  Uind : Gain  Gain=Unom/(2*pi*fnom)*sqrt(2)
  Unit Delay : UnitDelay  SampleTime=-1  HasFrameUpgradeWarning=on
  Unit Delay1 : UnitDelay  InitialCondition=gstart*65536*32768/180  SampleTime=TstepHw  HasFrameUpgradeWarning=on
  Vec3_y3_FB : libVishia_Conv/Vec3_y3_FB  SystemSampleTime=-1
  Vector Concatenate1 : Concatenate  NumInputs=3
  int32_radd_FB1 : libVishia_Conv/int32_radd_FB1  SystemSampleTime=-1
  rad_int32_FB : libVishia_Conv/rad_int32_FB  SystemSampleTime=-1
  rst_ab_FB : libVishia_Conv/rst_ab_FB  SystemSampleTime=-1
  scalar_Conv : libVishia_Conv/scalar_Conv  SystemSampleTime=-1
  xUI3mess : $bdroot/xUI3mess  SystemSampleTime=-1
  R : PMIOPort  Tag=PMCPort  Side=Right
  S : PMIOPort  Tag=PMCPort  Port=2  Side=Right
  T : PMIOPort  Tag=PMCPort  Port=3  Side=Right
  N : PMIOPort  Tag=PMCPort  Port=4  Side=Right
  Ik : Outport  OutDataTypeStr=double  PortDimensions=3
  Ui : Outport  Port=2
  Grotor : Outport  Port=3  OutDataTypeStr=int32  PortDimensions=1
  Gfq_rotor : Outport  Port=4  PortDimensions=1
  Hi : Outport  Port=5
  Pi : Outport  Port=6  OutDataTypeStr=double  PortDimensions=4
  Grotor1 : Outport  Port=7  OutDataTypeStr=double
  Out4 : Outport  Port=8  OutDataTypeStr=double
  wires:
  Constant1/1 -> Magnitude-Angle to Complex1/1
  rst_ab_FB/1 -> Unit Delay/1
  Damping/4(Out4) -> Out4/1  "Brotor"
  Damping/1(Out3) -> Sum3/1, Mux1/3
  Complex to Real-Imag1/1 -> DT1_FB/1
  Hiw/1 -> Gain3/1  "H_Ik"
  Gain2/1 -> Scope1/4, Mux/4, Product5/1, Product2/1, Vector Concatenate1/1, Scope2/1, Damping/1(In1)
  Product1/1 -> Mux/1, Scope1/1, Sum2/2
  Pmech/1 -> Mux1/1, Sum3/3  "Pmech"
  Sum1/1 -> Unit Delay1/1
  Unit Delay1/1 -> int32_radd_FB1/1, Grotor/1, Sum1/2  "Grotor"
  Gain/1 -> rad_int32_FB/1
  rad_int32_FB/1 -> Sum1/1
  Rotor/1 -> Rate Transition8/1  "Gfq_rotor"
  Demux/1 -> UemkR/1
  Sum2/1 -> Gain2/1  "Hsum"
  Uind/1 -> Demux/1, Mux2/1, Product/2, Scope/3  "Uind"
  Mux/1 -> Hi/1  "Hi"
  xUI3mess/2 -> Ik/1, Product/1, Scope/2, rst_ab_FB/1  "Ik"
  Unit Delay/1 -> Hiw/1
  Sum3/1 -> Hiw2/1, Mux1/4  "Psum"
  Gain5/1 -> Sum3/2, Mux1/2  "Pelec"
  Product/1 -> Scope/4, Vec3_y3_FB/1  "Pelec"
  Mux2/1 -> Ui/1
  Mux1/1 -> Pi/1
  Rate Transition8/1 -> Data Type Conversion3/1, Gain/1
  Data Type Conversion3/1 -> Gfq_rotor/1
  Hiw2/1 -> Rotor/1
  DT1_FB/2 -> Uind/1
  nHrotor/1 -> Product1/1  "nHrotor"
  Hrotor/1 -> Product1/2  "Hrotor"
  Damping/2(Out1) -> Mux/3, Scope1/3, Sum2/3
  Damping/3(Out2) -> Grotor1/1  "BIdamp"
  xUI3mess/1 -> Scope/1, Mux2/2
  Demux/2 -> UemkS/1
  Demux/3 -> UemkT/1
  Vec3_y3_FB/1 -> Add/1
  Vec3_y3_FB/2 -> Add/2
  Vec3_y3_FB/3 -> Add/3
  Add/1 -> Gain5/1
  Magnitude-Angle to Complex1/1 -> scalar_Conv/1
  int32_radd_FB1/1 -> Damping/2(In3), Magnitude-Angle to Complex1/2
  Gain3/1 -> Sum2/1, Mux/2, Scope1/2  "Hrotor"
  Constant4/1 -> Magnitude-Angle to Complex3/2
  Magnitude-Angle to Complex2/1 -> Product5/2
  Constant8/1 -> Magnitude-Angle to Complex2/1, Magnitude-Angle to Complex3/1
  Constant3/1 -> Magnitude-Angle to Complex2/2
  Magnitude-Angle to Complex3/1 -> Product2/2
  Product2/1 -> Scope2/3, Vector Concatenate1/3
  Product5/1 -> Vector Concatenate1/2, Scope2/2
  Vector Concatenate1/1 -> Complex to Real-Imag1/1
  scalar_Conv/1 -> Hrotor/1
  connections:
  N/RConn1 -- UemkS/LConn1 -- UemkR/LConn1 -- xUI3mess/LConn1 -- UemkT/LConn1
  UemkR/RConn1 -- Three-Phase Series RLC Branch/LConn1
  Three-Phase Series RLC Branch/LConn2 -- UemkS/RConn1
  Three-Phase Series RLC Branch/LConn3 -- UemkT/RConn1
  Three-Phase Series RLC Branch/RConn1 -- xUI3mess/LConn2
  Three-Phase Series RLC Branch/RConn2 -- xUI3mess/LConn3
  Three-Phase Series RLC Branch/RConn3 -- xUI3mess/LConn4
  xUI3mess/RConn1 -- R/RConn1
  xUI3mess/RConn2 -- S/RConn1
  xUI3mess/RConn3 -- T/RConn1

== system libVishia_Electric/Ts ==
  In1 : Inport  OutDataTypeStr=single
  Data Type Conversion : DataTypeConversion  OutDataTypeStr=single
  Data Type Conversion1 : DataTypeConversion  OutDataTypeStr=double
  Gain : Gain  Gain=1/Ts
  Integrator : Integrator
  Sum : Sum  Inputs=|+-
  Out1 : Outport  OutDataTypeStr=single
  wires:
  Sum/1 -> Gain/1
  Integrator/1 -> Data Type Conversion/1, Sum/2
  In1/1 -> Data Type Conversion1/1  "u"
  Gain/1 -> Integrator/1
  Data Type Conversion/1 -> Out1/1  "y"
  Data Type Conversion1/1 -> Sum/1

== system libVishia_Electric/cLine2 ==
  In1 : Inport
  Abs : Abs
  Constant : Constant  Value=xh
  Divide : Product  Inputs=*/
  Gain : Gain  Gain=n0*xh
  Gain1 : Gain  Gain=1-n2
  Sum : Sum  Inputs=|++
  Out1 : Outport
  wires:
  Divide/1 -> Out1/1  "y"
  Gain1/1 -> Sum/1
  In1/1 -> Abs/1, Gain/1  "u"
  Sum/1 -> Divide/2
  Constant/1 -> Sum/2
  Gain/1 -> Divide/1
  Abs/1 -> Gain1/1

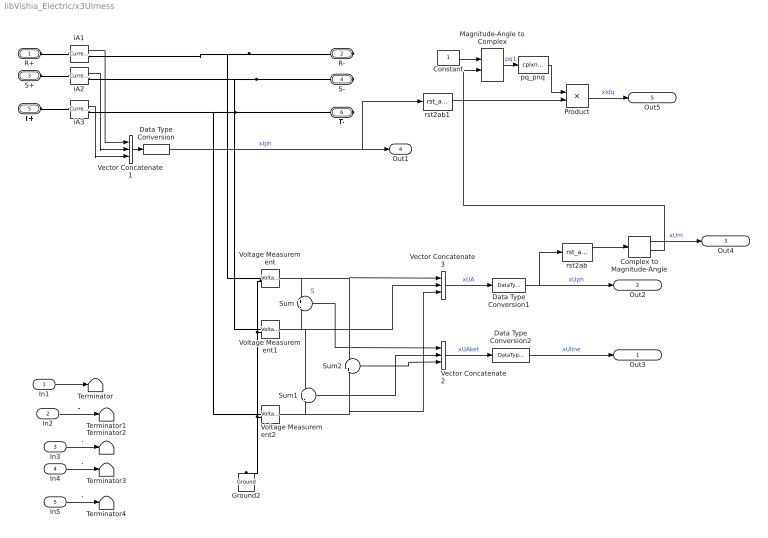
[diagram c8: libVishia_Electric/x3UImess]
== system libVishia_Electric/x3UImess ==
  note: S
  In1 : Inport
  In2 : Inport  Port=2
  In3 : Inport  Port=3
  In4 : Inport  Port=4
  In5 : Inport  Port=5
  Complex to Magnitude-Angle : ComplexToMagnitudeAngle
  Constant : Constant  OutDataTypeStr=single
  Data Type Conversion : DataTypeConversion  OutDataTypeStr=single
  Data Type Conversion1 : DataTypeConversion  OutDataTypeStr=single
  Data Type Conversion2 : DataTypeConversion  OutDataTypeStr=single
  Ground2 : powerlib/Elements/Ground  LConnTagsString=a
  Magnitude-Angle to Complex : MagnitudeAngleToComplex
  Product : Product
  Sum : Sum  Inputs=+|-
  Sum1 : Sum  Inputs=+|-
  Sum2 : Sum  Inputs=-|+
  Terminator{,1..4} (5 alike) : Terminator
  Vector Concatenate1 : Concatenate  NumInputs=3
  Vector Concatenate2 : Concatenate  NumInputs=3
  Vector Concatenate3 : Concatenate  NumInputs=3
  Voltage Measurement : powerlib/Measurements/Voltage Measurement  PhasorSimulation=off  OutputType=Complex  PSBequivalent=0
  Voltage Measurement1 : powerlib/Measurements/Voltage Measurement  PhasorSimulation=off  OutputType=Complex  PSBequivalent=0
  Voltage Measurement2 : powerlib/Measurements/Voltage Measurement  PhasorSimulation=off  OutputType=Complex  PSBequivalent=0
  iA1 : powerlib/Measurements/Current Measurement  PhasorSimulation=off  OutputType=Complex  PSBequivalent=0
  iA2 : powerlib/Measurements/Current Measurement  PhasorSimulation=off  OutputType=Complex  PSBequivalent=0
  iA3 : powerlib/Measurements/Current Measurement  PhasorSimulation=off  OutputType=Complex  PSBequivalent=0
  pq_pnq : libVishia_Conv/cplxni_FB  SystemSampleTime=-1
  rst2ab : libVishia_Conv/rst_ab_FB  SystemSampleTime=-1
  rst2ab1 : libVishia_Conv/rst_ab_FB  SystemSampleTime=-1
  R+ : PMIOPort  Side=Left
  R- : PMIOPort  Port=2  Side=Right
  S+ : PMIOPort  Port=3  Side=Left
  S- : PMIOPort  Port=4  Side=Right
  T+ : PMIOPort  Port=5  Side=Left
  T- : PMIOPort  Port=6  Side=Right
  Out3 : Outport
  Out2 : Outport  Port=2
  Out4 : Outport  Port=3
  Out1 : Outport  Port=4  OutDataTypeStr=single  PortDimensions=3
  Out5 : Outport  Port=5  OutDataTypeStr=single
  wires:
  Data Type Conversion/1 -> Out1/1, rst2ab1/1  "xIph"
  Vector Concatenate1/1 -> Data Type Conversion/1
  iA3/1 -> Vector Concatenate1/3
  iA2/1 -> Vector Concatenate1/2
  iA1/1 -> Vector Concatenate1/1
  Sum2/1 -> Vector Concatenate2/3
  Sum1/1 -> Vector Concatenate2/2
  Sum/1 -> Vector Concatenate2/1
  Data Type Conversion2/1 -> Out3/1  "xUline"
  Vector Concatenate2/1 -> Data Type Conversion2/1  "xUAket"
  Data Type Conversion1/1 -> rst2ab/1, Out2/1  "xUph"
  Vector Concatenate3/1 -> Data Type Conversion1/1  "xUA"
  Voltage Measurement2/1 -> Vector Concatenate3/3, Sum2/2, Sum1/2
  Voltage Measurement1/1 -> Vector Concatenate3/2, Sum1/1, Sum/2
  Voltage Measurement/1 -> Sum2/1, Vector Concatenate3/1, Sum/1
  In1/1 -> Terminator/1  "-"
  In2/1 -> Terminator1/1  "-"
  In3/1 -> Terminator2/1  "-"
  rst2ab/1 -> Complex to Magnitude-Angle/1
  Complex to Magnitude-Angle/1 -> Out4/1  "xUm"
  pq_pnq/1 -> Product/1
  Complex to Magnitude-Angle/2 -> Magnitude-Angle to Complex/2
  rst2ab1/1 -> Product/2
  Product/1 -> Out5/1  "xIdq"
  In4/1 -> Terminator3/1  "-"
  In5/1 -> Terminator4/1  "-"
  Constant/1 -> Magnitude-Angle to Complex/1
  Magnitude-Angle to Complex/1 -> pq_pnq/1  "pq1"
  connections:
  T+/RConn1 -- iA3/LConn1
  S+/RConn1 -- iA2/LConn1
  R+/RConn1 -- iA1/LConn1
  T-/RConn1 -- Voltage Measurement2/LConn1 -- iA3/RConn1
  S-/RConn1 -- Voltage Measurement1/LConn1 -- iA2/RConn1
  R-/RConn1 -- Voltage Measurement/LConn1 -- iA1/RConn1
  Voltage Measurement/LConn2 -- Voltage Measurement1/LConn2 -- Ground2/LConn1 -- Voltage Measurement2/LConn2

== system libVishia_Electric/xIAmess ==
  Data Type Conversion : DataTypeConversion  OutDataTypeStr=single
  Vector Concatenate1 : Concatenate  NumInputs=3
  iA1 : powerlib/Measurements/Current Measurement  PhasorSimulation=off  OutputType=Complex  PSBequivalent=0
  iA2 : powerlib/Measurements/Current Measurement  PhasorSimulation=off  OutputType=Complex  PSBequivalent=0
  iA3 : powerlib/Measurements/Current Measurement  PhasorSimulation=off  OutputType=Complex  PSBequivalent=0
  R+ : PMIOPort  Side=Left
  R- : PMIOPort  Port=2  Side=Right
  S+ : PMIOPort  Port=3  Side=Left
  S- : PMIOPort  Port=4  Side=Right
  T+ : PMIOPort  Port=5  Side=Left
  T- : PMIOPort  Port=6  Side=Right
  Out1 : Outport  OutDataTypeStr=single  PortDimensions=3
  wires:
  iA1/1 -> Vector Concatenate1/1
  iA2/1 -> Vector Concatenate1/2
  iA3/1 -> Vector Concatenate1/3
  Vector Concatenate1/1 -> Data Type Conversion/1
  Data Type Conversion/1 -> Out1/1  "xIrst"
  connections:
  R-/RConn1 -- iA1/RConn1
  S-/RConn1 -- iA2/RConn1
  T-/RConn1 -- iA3/RConn1
  R+/RConn1 -- iA1/LConn1
  S+/RConn1 -- iA2/LConn1
  T+/RConn1 -- iA3/LConn1

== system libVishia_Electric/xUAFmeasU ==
  note: S
  Data Type Conversion : DataTypeConversion  OutDataTypeStr=single
  Data Type Conversion1 : DataTypeConversion  OutDataTypeStr=single
  Ground2 : powerlib/Elements/Ground  LConnTagsString=a
  Sum : Sum  Inputs=+|-
  Sum1 : Sum  Inputs=+|-
  Sum2 : Sum  Inputs=-|+
  Vector Concatenate1 : Concatenate  NumInputs=3
  Vector Concatenate2 : Concatenate  NumInputs=3
  Voltage Measurement : powerlib/Measurements/Voltage Measurement  PhasorSimulation=off  OutputType=Complex  PSBequivalent=0
  Voltage Measurement1 : powerlib/Measurements/Voltage Measurement  PhasorSimulation=off  OutputType=Complex  PSBequivalent=0
  Voltage Measurement2 : powerlib/Measurements/Voltage Measurement  PhasorSimulation=off  OutputType=Complex  PSBequivalent=0
  Conn1 : PMIOPort  Side=Left
  Conn2 : PMIOPort  Port=2  Side=Left
  Conn3 : PMIOPort  Port=3  Side=Left
  Out2 : Outport
  Out1 : Outport  Port=2
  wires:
  Voltage Measurement/1 -> Sum/1, Vector Concatenate2/1, Sum2/1
  Voltage Measurement1/1 -> Sum/2, Sum1/1, Vector Concatenate2/2
  Voltage Measurement2/1 -> Sum1/2, Sum2/2, Vector Concatenate2/3
  Vector Concatenate2/1 -> Data Type Conversion/1  "xUA"
  Data Type Conversion/1 -> Out2/1  "xUphase"
  Vector Concatenate1/1 -> Data Type Conversion1/1  "xUAket"
  Data Type Conversion1/1 -> Out1/1  "xUket"
  Sum/1 -> Vector Concatenate1/1
  Sum1/1 -> Vector Concatenate1/2
  Sum2/1 -> Vector Concatenate1/3
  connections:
  Voltage Measurement/LConn1 -- Conn1/RConn1  "R"
  Voltage Measurement2/LConn1 -- Conn3/RConn1  "T"
  Voltage Measurement/LConn2 -- Voltage Measurement2/LConn2 -- Ground2/LConn1 -- Voltage Measurement1/LConn2
  Voltage Measurement1/LConn1 -- Conn2/RConn1  "S"

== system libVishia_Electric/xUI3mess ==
  In2 : Inport
  Current Measurement : powerlib/Measurements/Current Measurement  PhasorSimulation=off  OutputType=Complex  PSBequivalent=0
  Current Measurement1 : powerlib/Measurements/Current Measurement  PhasorSimulation=off  OutputType=Complex  PSBequivalent=0
  Current Measurement2 : powerlib/Measurements/Current Measurement  PhasorSimulation=off  OutputType=Complex  PSBequivalent=0
  Terminator1 : Terminator
  Uk : powerlib/Measurements/Voltage Measurement  PhasorSimulation=off  OutputType=Complex  PSBequivalent=0
  Uk2 : powerlib/Measurements/Voltage Measurement  PhasorSimulation=off  OutputType=Complex  PSBequivalent=0
  Uk3 : powerlib/Measurements/Voltage Measurement  PhasorSimulation=off  OutputType=Complex  PSBequivalent=0
  Vector Concatenate : Concatenate  NumInputs=3
  Vector Concatenate2 : Concatenate  NumInputs=3
  N : PMIOPort  Side=Left
  R1 : PMIOPort  Port=2  Side=Left
  R2 : PMIOPort  Port=3  Side=Right
  S1 : PMIOPort  Port=4  Side=Left
  S2 : PMIOPort  Port=5  Side=Right
  T1 : PMIOPort  Port=6  Side=Left
  T2 : PMIOPort  Port=7  Side=Right
  Uk1 : Outport  OutDataTypeStr=double  PortDimensions=3
  Uk5 : Outport  Port=2  OutDataTypeStr=double  PortDimensions=3
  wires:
  Uk/1 -> Vector Concatenate/1  "Uk"
  Vector Concatenate/1 -> Uk1/1  "U"
  Uk2/1 -> Vector Concatenate/2  "Uk"
  Uk3/1 -> Vector Concatenate/3  "Uk"
  Vector Concatenate2/1 -> Uk5/1  "I"
  Current Measurement/1 -> Vector Concatenate2/1
  Current Measurement1/1 -> Vector Concatenate2/2
  Current Measurement2/1 -> Vector Concatenate2/3
  In2/1 -> Terminator1/1  "-"
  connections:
  Uk/LConn1 -- R1/RConn1 -- Current Measurement/LConn1
  R2/RConn1 -- Current Measurement/RConn1
  Current Measurement1/LConn1 -- S1/RConn1 -- Uk2/LConn1
  S2/RConn1 -- Current Measurement1/RConn1
  Current Measurement2/LConn1 -- T1/RConn1 -- Uk3/LConn1
  T2/RConn1 -- Current Measurement2/RConn1
  N/RConn1 -- Uk3/LConn2 -- Uk2/LConn2 -- Uk/LConn2
